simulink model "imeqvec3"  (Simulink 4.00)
settings: Solver=ode45  StartTime=0.0  StopTime=1  MaxStep=1e-3  RelTol=1e-3
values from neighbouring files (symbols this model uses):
  H = 0.60    (= 0.6)    [IMabc2.m]    (also in IMcur0.m = 0.3; imdef0vec.m = 0.3; imdef1vec.m = 0.3; imdef2vec.m = 0.3)
  ic = [fs0 fr0]    [imdef0vec.m]    (also in imdef1vec.m; imdef2vec.m = F; imic2.m = [phids phiqs phidr phiqr n0]'; imic3.m = [phids phiqs phidr phiqr n0]')
  Lm = eval(get(hLm,'String'))    [im3d.m]    (also in IMabc2.m = 4.5; imabcparam.m = 0.0847; IMabcrun0.m = 0.0847; IMabcrun1.m = 0.0847)
  Lrl = eval(get(hLr,'String'))    [im3d.m]    (also in IMabc2.m = 0.1; imabcparam.m = 0.0025; IMabcrun0.m = 0.0025; IMabcrun1.m = 0.0025)
  Lsl = eval(get(hLs,'String'))    [im3d.m]    (also in IMabc2.m = 0.1; imabcparam.m = 0.0025; IMabcrun0.m = 0.0025; IMabcrun1.m = 0.0025)
  n0 = 0.98    [imdef0vec.m]    (also in imdef1vec.m = 0.978; imdef2vec.m; imdefrotflux.m; imdefSIvec1.m = 0.95)
  Rr = input('Rotor resistance)[default = 2] =')    [Actac.m]    (also in im1phase.m = 0.3; im3d.m = eval(get(hRr,'String')); IMabc2.m = 0.02; imabcparam.m = 0.408)
  Rs = eval(get(hRs,'String'))    [im3d.m]    (also in IMabc2.m = 0.01; imabcparam.m = 0.531; IMabcrun0.m = 0.531; IMabcrun1.m = 0.531)
  Tl0 = Is*conj(Is)*Req    [imdef0vec.m]    (also in imdef1vec.m; imdef2vec.m = Lm*(I(2)*I(3)-I(1)*I(4)); imdefrotflux.m; imdefSIvec1.m = Te0/To)
  vs = 1.0    (= 1)    [imdef0vec.m]    (also in imdef1vec.m; imdef2vec.m; imdefrotflux.m; imdefSIvec1.m)
  wk = ws    (= 1)    [imdef0vec.m]    (also in imdef1vec.m; imdef2vec.m; imdefrotflux.m; imdefSIvec1.m)
  wo = 2*pi*freq0    [calc0.m]    (also in IMabc2.m = 376.991118431; imabcparam.m = 376.991118431; IMabcrun0.m = 376.991118431; IMabcrun1.m = 376.991118431)

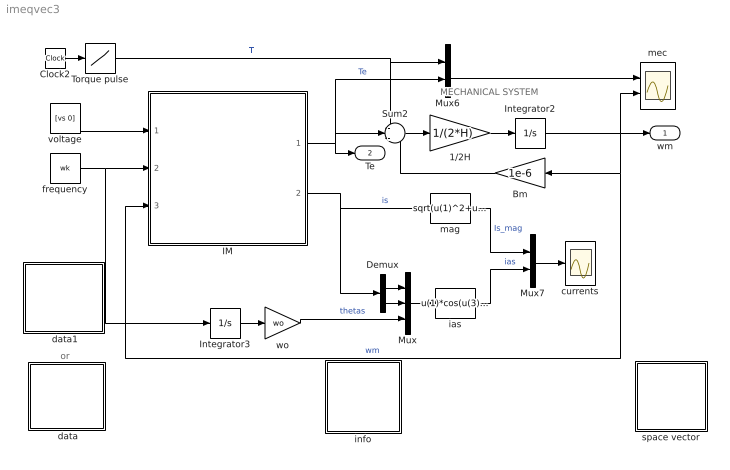
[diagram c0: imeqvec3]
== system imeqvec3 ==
  note: or
  note: MECHANICAL SYSTEM
  " data" : Subsystem
  " data1" : Subsystem
  1/2H : Gain  Gain=1/(2*H)  Multiplication=Element-wise(K.*u)  SaturateOnIntegerOverflow=on
  Bm : Gain  Orientation=left  Gain=1e-6  Multiplication=Element-wise(K.*u)  SaturateOnIntegerOverflow=on
  Clock2 : Clock
  Demux : Demux  Outputs=2  BusSelectionMode=off
  IM : Subsystem
  Integrator2 : Integrator  ExternalReset=none  InitialConditionSource=internal  InitialCondition=n0  LimitOutput=off  UpperSaturationLimit=inf  LowerSaturationLimit=-inf  ShowSaturationPort=off  ShowStatePort=off  AbsoluteTolerance=auto
  Integrator3 : Integrator  ExternalReset=none  InitialConditionSource=internal  InitialCondition=0  LimitOutput=off  UpperSaturationLimit=inf  LowerSaturationLimit=-inf  ShowSaturationPort=off  ShowStatePort=off  AbsoluteTolerance=auto
  Mux : Mux  Inputs=3
  Mux6 : Mux  Inputs=2
  Mux7 : Mux  Inputs=2
  Sum2 : Sum  Inputs=-+-  SaturateOnIntegerOverflow=on
  Torque pulse : Lookup  InputValues=[0 0.1 0.1 0.5 0.5 2]  OutputValues="[Tl0 Tl0  0 0 0.5 0.5]"
  currents : Scope
  frequency : Constant  Value=wk
  ias : Fcn  Expr=u(1)*cos(u(3))-u(2)*sin(u(3))
  info : Subsystem
  mag : Fcn  Expr=sqrt(u(1)^2+u(2)^2)
  mec : Scope  NumInputPorts=2
  space vector : Subsystem
  voltage : Constant  Value=[vs 0]
  wo : Gain  Gain=wo  Multiplication=Element-wise(K.*u)  SaturateOnIntegerOverflow=on
  wm : Outport  Port=1
  Te : Outport  Port=2
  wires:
  voltage/1 -> IM/1(vs)
  frequency/1 -> Integrator3/1, IM/2(wk)
  Demux/1 -> Mux/1
  Demux/2 -> Mux/2
  Mux/1 -> ias/1
  ias/1 -> Mux7/2  "ias"
  mag/1 -> Mux7/1  "Is_mag"
  Mux7/1 -> currents/1
  IM/2(is) -> mag/1, Demux/1  "is"
  Sum2/1 -> 1/2H/1
  1/2H/1 -> Integrator2/1
  Mux6/1 -> mec/1
  IM/1(Te) -> Sum2/2, Mux6/2, Te/1  "Te"
  Bm/1 -> Sum2/3
  Integrator3/1 -> wo/1
  wo/1 -> Mux/3  "thetas"
  Integrator2/1 -> mec/2, wm/1, IM/3(wm), Bm/1  "wm"
  Clock2/1 -> Torque pulse/1
  Torque pulse/1 -> Mux6/1, Sum2/1  "Tl"

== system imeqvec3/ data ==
  note: This demo simulates the running of an induction motor in steady-state when a sudden input change is effected: a)torque step changes at constant voltage excitation b) voltage input sag at constant frequency and load torque c)simultaneous step changes in voltage magnitude and frequency
  note: Double click the block to enter the machine parameters and initial conditions and then run the simulation

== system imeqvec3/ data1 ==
  note: This demo simulates the running of an induction motor in steady-state when a sudden input change is effected: a)torque step changes at constant voltage excitation b) voltage input sag at constant frequency and load torque c)simultaneous step changes in voltage magnitude and frequency
  note: Double click the block to enter the machine parameters and initial conditions and then run the simulation

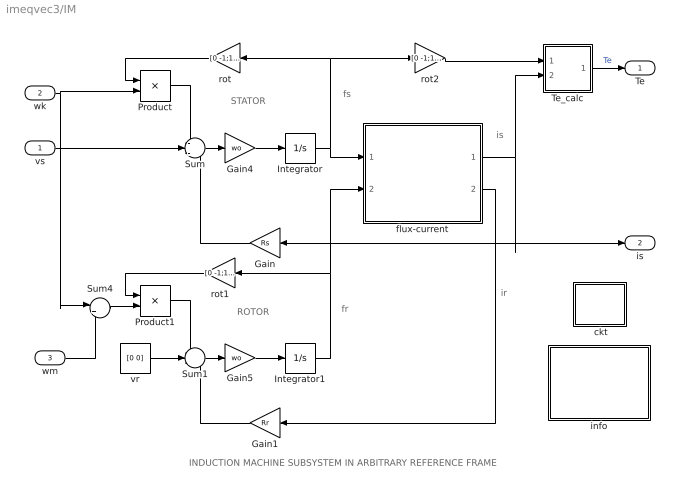
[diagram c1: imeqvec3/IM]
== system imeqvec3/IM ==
  note: ROTOR
  note: STATOR
  note: fs
  note: fr
  note: is
  note: INDUCTION MACHINE SUBSYSTEM IN ARBITRARY REFERENCE FRAME
  note: ir
  vs : Inport  Port=1
  wk : Inport  Port=2
  wm : Inport  Port=3
  " ckt" : Subsystem
  Gain : Gain  Orientation=left  Gain=Rs  Multiplication=Element-wise(K.*u)  SaturateOnIntegerOverflow=on
  Gain1 : Gain  Orientation=left  Gain=Rr  Multiplication=Element-wise(K.*u)  SaturateOnIntegerOverflow=on
  Gain4 : Gain  Gain=wo  Multiplication=Element-wise(K.*u)  SaturateOnIntegerOverflow=on
  Gain5 : Gain  Gain=wo  Multiplication=Element-wise(K.*u)  SaturateOnIntegerOverflow=on
  Integrator : Integrator  ExternalReset=none  InitialConditionSource=internal  InitialCondition=[ic(1) ic(2)]  LimitOutput=off  UpperSaturationLimit=inf  LowerSaturationLimit=-inf  ShowSaturationPort=off  ShowStatePort=off  AbsoluteTolerance=auto
  Integrator1 : Integrator  ExternalReset=none  InitialConditionSource=internal  InitialCondition=[ic(3) ic(4)]  LimitOutput=off  UpperSaturationLimit=inf  LowerSaturationLimit=-inf  ShowSaturationPort=off  ShowStatePort=off  AbsoluteTolerance=auto
  Product : Product  Inputs=2  Multiplication=Element-wise(.*)  SaturateOnIntegerOverflow=on
  Product1 : Product  Inputs=2  Multiplication=Element-wise(.*)  SaturateOnIntegerOverflow=on
  Sum : Sum  Inputs=-+-  SaturateOnIntegerOverflow=on
  Sum1 : Sum  Inputs=-+-  SaturateOnIntegerOverflow=on
  Sum4 : Sum  Inputs=|+-  SaturateOnIntegerOverflow=on
  Te_calc : Subsystem
  flux-current : Subsystem
  info : Subsystem
  rot : Gain  Orientation=left  Gain=[0 -1;1 0]  Multiplication=Matrix(K*u)  SaturateOnIntegerOverflow=on
  rot1 : Gain  Orientation=left  Gain=[0 -1;1 0]  Multiplication=Matrix(K*u)  SaturateOnIntegerOverflow=on
  rot2 : Gain  Gain=[0 -1;1 0]  Multiplication=Matrix(K*u)  SaturateOnIntegerOverflow=on
  vr : Constant  Value=[0 0]
  Te : Outport  Port=1
  is : Outport  Port=2
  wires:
  Gain/1 -> Sum/3
  vr/1 -> Sum1/2
  Gain1/1 -> Sum1/3
  Integrator/1 -> flux-current/1(fs), rot/1, rot2/1
  Integrator1/1 -> flux-current/2(fr), rot1/1
  Product1/1 -> Sum1/1
  rot1/1 -> Product1/1
  Product/1 -> Sum/1
  rot/1 -> Product/1
  rot2/1 -> Te_calc/1(fs)
  Sum4/1 -> Product1/2
  Sum/1 -> Gain4/1
  Gain4/1 -> Integrator/1
  Sum1/1 -> Gain5/1
  Gain5/1 -> Integrator1/1
  flux-current/1(is) -> Te_calc/2(is), Gain/1, is/1
  Te_calc/1(Te) -> Te/1  "Te"
  vs/1 -> Sum/2
  wk/1 -> Product/2, Sum4/1
  wm/1 -> Sum4/2
  flux-current/2(ir) -> Gain1/1

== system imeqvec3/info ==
  note: The induction machine is modeled in vectorized form in conformity with the state vector formulation. This one-to-one correspondence can be seen by clicking both the INDUCTION MACHINE subsystem block and the MATHEMATICAL MODEL equation block. The synchronous reference frame is chosen here because the machine is operating under balanced three-phase sinusoidal excitation; the input voltage is thefore constant as indicated. The parameters describing the electromechanical system are expressed in per unit and are entered after double-clicking one of the PARAMETERS/IC blocks. The system is initially assumed to be operated under load in a steady state defined by a specified speed. The initial conditions are established by calling a phasor calculation based on the standard steady-state equivalent circuit of the induction machine. The simulation can then be run. In the present case, it exhibits the dynamic response to a pulsed applied torque. The torque developed, the speed, and the stator current are observed on the scopes . The torque-speed dynamic characteristics can then be obtained after double clicking the X-Y PLOT block.
  note: Running of a Line-Fed Induction Motor Synchronous frame Per unit system

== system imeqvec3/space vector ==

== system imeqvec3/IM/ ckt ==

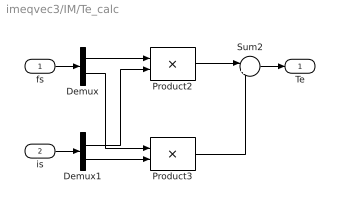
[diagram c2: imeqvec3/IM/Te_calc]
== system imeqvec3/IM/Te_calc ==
  fs : Inport  Port=1
  is : Inport  Port=2
  Demux : Demux  Outputs=2  BusSelectionMode=off
  Demux1 : Demux  Outputs=2  BusSelectionMode=off
  Product2 : Product  Inputs=2  Multiplication=Element-wise(.*)  SaturateOnIntegerOverflow=on
  Product3 : Product  Inputs=2  Multiplication=Element-wise(.*)  SaturateOnIntegerOverflow=on
  Sum2 : Sum  Inputs=|++  SaturateOnIntegerOverflow=on
  Te : Outport  Port=1
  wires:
  Demux/1 -> Product2/1
  Demux1/2 -> Product3/2
  Demux/2 -> Product3/1
  Demux1/1 -> Product2/2
  Product2/1 -> Sum2/1
  Product3/1 -> Sum2/2
  Sum2/1 -> Te/1
  fs/1 -> Demux/1
  is/1 -> Demux1/1

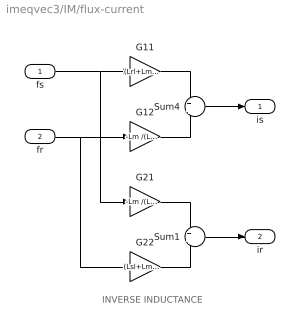
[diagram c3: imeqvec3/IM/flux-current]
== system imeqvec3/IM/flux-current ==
  note: INVERSE INDUCTANCE
  fs : Inport  Port=1
  fr : Inport  Port=2
  G11 : Gain  Gain=(Lrl+Lm) /(Lsl*Lrl+Lsl*Lm+Lrl*Lm)  Multiplication=Element-wise(K.*u)  SaturateOnIntegerOverflow=on
  G12 : Gain  Gain=-Lm /(Lsl*Lrl+Lsl*Lm+Lrl*Lm)  Multiplication=Element-wise(K.*u)  SaturateOnIntegerOverflow=on
  G21 : Gain  Gain=-Lm /(Lsl*Lrl+Lsl*Lm+Lrl*Lm)  Multiplication=Element-wise(K.*u)  SaturateOnIntegerOverflow=on
  G22 : Gain  Gain=(Lsl+Lm )/(Lsl*Lrl+Lsl*Lm+Lrl*Lm)  Multiplication=Element-wise(K.*u)  SaturateOnIntegerOverflow=on
  Sum1 : Sum  Inputs=++  SaturateOnIntegerOverflow=on
  Sum4 : Sum  Inputs=++  SaturateOnIntegerOverflow=on
  is : Outport  Port=1
  ir : Outport  Port=2
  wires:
  fs/1 -> G11/1, G21/1
  G11/1 -> Sum4/1
  fr/1 -> G12/1, G22/1
  G12/1 -> Sum4/2
  Sum4/1 -> is/1
  G21/1 -> Sum1/1
  G22/1 -> Sum1/2
  Sum1/1 -> ir/1

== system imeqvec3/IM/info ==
  note: Mathematical model of the induction machine. Space vector formulation in an arbitrary dq common reference frame. Per unit description.
  note: Electrical system equations: vs = Rs is + 1/wo (dfs/dt) + wk M(pi/2) fs vr = Rr ir + 1/wo (dfr/dt) + (wk - wm) M(pi/2) fr where the variables i, v, and f are 2-dimensional space vectors; for instance is = [ids iqs] and so forth, wk is the speed of the reference frame, wm the rotor speed, and M(pi/2)represents a 90o space rotator namely M(pi/2) = [0 -1;1 0] The flux linkage current relations are: fds = Ls ids + Lm idr fdr = Lm ids + Lr idr (D_axis) Ls =Lm +Lsl ; Lr = Lm +Lrl fqs = Ls iqs + Lm iqr fqr = Lm iqs + Lr iqr (Q_axis) Mechanical system equations: Te = 2H (dwm/dt ) + Bm wm + Tl where Te = fs (cross) is = M(pi/2) fs (dot) is = fds iqs - fqs ids = fs x is = M(pi/2) fs . is = ir x fr = Lm (ir x is) = Lm/Lr (fr x is) = 1/Lm' (fr x fs) Lm' =Lm c/(1-c) c = 1 - Lm^2/(Ls Lr)
